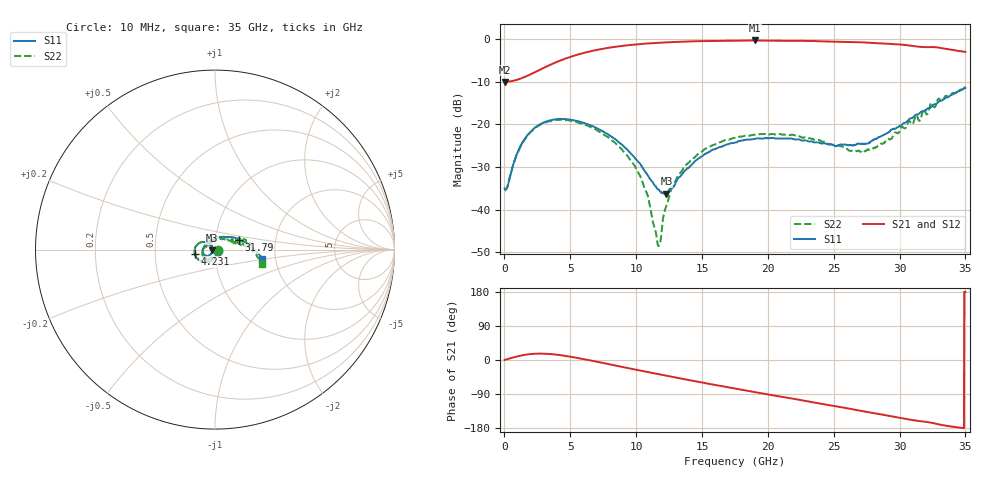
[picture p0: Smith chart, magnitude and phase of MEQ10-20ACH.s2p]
! MARKI MICROWAVE INC.
! Email:  support@markimicrowave.com  Phone:  408-778-4200
! Model Number:  MEQ10-20ACH  Date:  6/18
! Filename:		MEQ10-20ACH.S2P  Version: 1.0
! Description:  2-port S-parameter data for chip equalizer
! Features:		Low Insertion Loss, Excellent Return Loss
! Frequency Measured: 	10 MHz to 35 GHz
!S2P File: Measurements: S11, S21, S12, S22:
# Hz S  dB  R 50
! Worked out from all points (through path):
!   1601 points, 10 MHz to 35 GHz, reference 50 ohm
!   highest |S21| = -0.29 dB at 19.04 GHz (marker M1); lowest = -10.0 dB at 10 MHz (marker M2)
!   group delay of S21, straight-line fit = 17 ps
!   lowest |S11| = -36.2 dB at 12.3 GHz (marker M3), VSWR 1.03, Z = 48.5 - j0.355 ohm
!   |S11| at or under -10 dB: start of sweep to end of sweep
!   |S22| runs from -48.6 to -11.2 dB; largest |S21 - S12| = 0.0093
!   S11 on the Smith chart (normalised r, x): 10 MHz: 1.03, -0.01; 4.231 GHz: 0.80, -0.04; 31.79 GHz: 1.30, +0.14; 35 GHz: 1.70, -0.18
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1e7  -35.05 -21.9  -10.03 0.2  -10.05 0.6  -35.58 -13.8
2.505562e8  -34.37 -40.4  -9.95 2.6  -9.94 2.6  -34.36 -40.0
9.940938e8  -26.56 -93.2  -9.49 9.7  -9.48 9.7  -26.71 -92.8
1.781369e9  -22.40 -117.8  -8.52 14.8  -8.52 14.8  -22.50 -118.3
4.230669e9  -18.72 -168.6  -5.01 12.9  -5.01 12.9  -18.92 -170.2
5.848956e9  -19.50 167.6  -3.35 3.5  -3.35 3.5  -19.78 165.0
7.948356e9  -22.49 145.0  -1.99 -11.1  -1.99 -11.2  -23.20 139.7
9.829069e9  -27.60 134.9  -1.27 -24.6  -1.27 -24.5  -29.44 122.5
1.083503e10  -31.75 140.0  -1.00 -31.6  -1.00 -31.6  -36.30 120.6
1.168791e10  -35.27 161.7  -0.84 -37.5  -0.83 -37.5  -48.59 -153.9
1.181912e10  -35.72 167.4  -0.81 -38.4  -0.81 -38.4  -47.72 -134.5
1.230024e10  -36.24 -166.3  -0.74 -41.7  -0.73 -41.7  -39.03 -102.7
1.280322e10  -34.78 -148.5  -0.67 -45.0  -0.66 -45.0  -34.40 -101.1
1.380918e10  -30.57 -134.1  -0.54 -51.6  -0.55 -51.7  -29.47 -104.3
1.529626e10  -26.87 -134.5  -0.43 -61.4  -0.43 -61.3  -25.64 -113.9
1.7505e10  -24.22 -145.9  -0.35 -75.1  -0.34 -75.3  -23.17 -129.6
1.903581e10  -23.37 -157.4  -0.29 -84.8  -0.30 -84.7  -22.45 -140.3
2.334396e10  -24.02 163.8  -0.43 -111.1  -0.42 -111.0  -23.37 -177.1
2.717099e10  -24.55 98.7  -0.73 -134.8  -0.75 -134.6  -26.60 115.0
2.918291e10  -21.83 59.9  -1.07 -147.1  -1.05 -147.6  -23.37 64.5
3.178529e10  -16.95 21.4  -1.84 -162.2  -1.84 -161.8  -16.51 18.2
3.5e10  -11.42 -10.8  -2.97 179.5  -3.01 180.0  -11.20 -17.1
